(* Logix 5000 AddOnInstructionDefinition export Banner_QS18EAF_Param_v4; software revision 33.00 *)

TYPE Banner_IOL_Port_v4 :   // UDT that has all of the data items necessary to communicate with a specific Port on a IO-Link Master
STRUCT
   Port_Controlled : INT;   // Each bit represents a port on an IO-Link Master. Set to 1 to tell AOI to control that port.
   Port_Activate : INT;   // Each bit represents a port on an IO-Link Master. When ON that port will process any commands in queue.
   Port_Read : INT;   // Each bit represents a port on an IO-Link Master. Used to determine when device AOI has requested a Read command.
   Port_Write : INT;   // Each bit represents a port on an IO-Link Master. Used to determine when device AOI has requested a Write command.
   Port_RW_Complete : INT;   // Each bit represents a port on an IO-Link Master. Tells device AOI that Read or Write request has been completed.
   Port_Device_Read : INT;
   Data_Transfer : SINT[190];   // Array to transfer data from IO-Master to device AOIs.
END_STRUCT
END_TYPE

TYPE Banner_QS18EAF_RD_v4 :   // UDT that stores the Write Data for a QS18EAF.
STRUCT
   Master_Cycle_Time : INT;
   Min_Cycle_Time : INT;
   M_Sequence_Capability : INT;
   IO_Link_Version_ID : INT;
   Process_Data_Input_Length : INT;
   Process_Data_Output_Length : INT;
   Combined_Vendor_ID : DINT;   // IO-Link Vendor ID
   Vendor_ID1 : INT;
   Vendor_ID2 : INT;
   Combined_Device_ID : DINT;   // IO-Link Device ID
   Device_ID1 : INT;
   Device_ID2 : INT;
   Device_ID3 : INT;
   Serial_Number : STRING;
   Teach_State : SINT;   // 0 = Idle, 1 = SP1 Success, 4 = Wait for Command, 5 = Busy, 6 = Error.
   SP_TP1 : SINT;
   SP_TP2 : SINT;
   Current_Setpoint : DINT;   // Value in .1mm increments.
   Taught_Status : SINT;   // 0 = Not taught, 1 = Taught, 2 = Coerced to near limit, 3 = Coerced to far limit.
   All_Time_Run_Time_Counter : DINT;   // 0 to 2 Billion. 1/4 hr increments.
END_STRUCT
END_TYPE

TYPE Banner_QS18EAF_v4 :   // All of the parameters for a QS18EAF.
STRUCT
   Initial_Global_Read : BOOL;   // Determines if all of the IO-Link data has been read into the PLC yet
   Command : INT;   // Value placed in here will activate a read or write to a specifc IO-Link Index
   Read_Data : Banner_QS18EAF_RD_v4;   // Read Only Data
   Write_Data : Banner_QS18EAF_WD_v4;   // Write Data
   Archive_Data : Banner_QS18EAF_WD_v4;   // Archive Data
   Reset : BOOL;   // Resets AOI. This will force a complete parameter read of the sensor.
END_STRUCT
END_TYPE

TYPE Banner_QS18EAF_WD_v4 :   // UDT that stores the Write Data for a QS18EAF.
STRUCT
   System_Command : INT;   // See IODD file for list of commands that can be activated via the System Command interface
   Parameter_Access_Lock : SINT;   // Write access to all parameters is prohibited while value is 1. Only this parameter can be adjusted when value is 1.
   Data_Storage_Lock : SINT;   // Automatic data storage is disabled when this value is equal to 1. Read access is not affected.
   Local_Parameterization_Lock : SINT;   // Parameterization via local control elements on device is disabled.
   Local_User_Interface_Lock : SINT;   // Operation of local user interface is disabled.
   BDC1_Setpoint_SP1 : INT;   // Setpoint value in .1 mm increments.
   BDC1_Setpoint_SP2 : INT;   // Unused must be written to 0.
   BDC1_Swithpoint_Logic : INT;   // 0 = Light Operate, 1 = Dark Operate
   BDC1_BDC_Mode : INT;   // 1 = 1-Pt BGS, 128 = Object Set. Defines how the binary switching information is created depending on Setpoint parameters (SP1, SP2) and the current measurement value.
   BDC1_Hysteresis : DINT;   // Should always be 0
   BDC1_BDC_Setpoint_Selection : SINT;   // 0 = Local 1 = Remote. Controls wheater the setpoint is controlled by the POT or via the value in SP1.
   BDC1_Delay_Mode : SINT;   // 0 = Disabled, 1 = On-Off Delay, 2 = Oneshot.
   BDC1_Delay_Timer_1 : DINT;   // Range 0 to 90000. On delay or Oneshot time.
   BDC1_Delay_Timer_2 : DINT;   // Range 0 to 90000. Off delay time. If oneshot mode active this must be written as 0.
   Teach_Offset_Mode : SINT;   // 0 = Auto, 1 = User. Select between automatic tach offset and value stored in user teach offset.
   User_Teach_Offset : INT;   // User select teach offset in .1 mm increments.
   Pin_2_Configuration : SINT;   // 0 = Detection Output, 1 = Complimentary Output.
   Response_Speed : INT;   // 0 = High Speed (450 microsecond On/Off), 1 = Cross-talk (1.1 ms On/Off), 2 = Robust (1.7 ms On; 1.1 ms Off).
   Resettable_Run_Time_Counter : DINT;   // 0 to 2 Billion. 1/4 hr increments.
   All_Time_Run_Time_Event_Time : DINT;   // 0 to 2 Billion. 1/4 hr increments.
   Resettable_Run_Time_Event_Time_Counter : DINT;   // 0 to 2 Billion. 1/4 hr increments.
END_STRUCT
END_TYPE

ADD_ON_INSTRUCTION Banner_QS18EAF_Param_v4   (* revision 4.0, vendor Banner Engineering *)
// AOI to read and write parameter data to an IO-Link QS18 EAF.
VAR_IN_OUT
   QS18EAF : Banner_QS18EAF_v4; {required}
   Port_Data : Banner_IOL_Port_v4; {required}
END_VAR
VAR_INPUT
   Port : DINT; {required}
END_VAR
VAR
   Local_Control : DINT; {access None}
   Global_Read_Command_Value : INT; {access None}
   Global_Write_Command_Value : INT; {access None}
   Command_Being_Processed : BOOL; {access None}
   Update_Archive : BOOL; {access None}
   Index_Write_Inprocess : INT; {access None}
   Index_Write_Control : INT; {access None}
   Inprocess_Index : DINT; {access None}
END_VAR

ROUTINE Logic   (* ladder *)
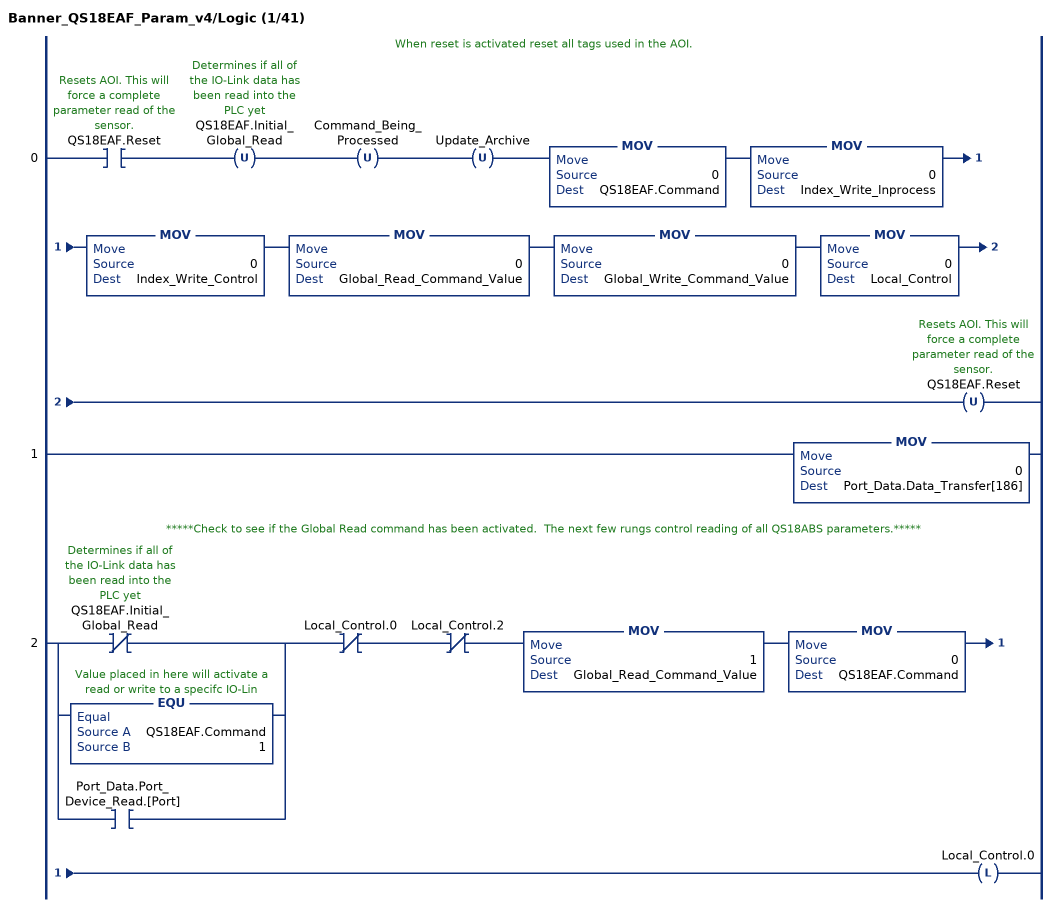
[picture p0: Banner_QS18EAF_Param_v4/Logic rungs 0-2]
   // When reset is activated reset all tags used in the AOI.
   0: XIC(QS18EAF.Reset)OTU(QS18EAF.Initial_Global_Read)OTU(Command_Being_Processed)OTU(Update_Archive)MOV(0,QS18EAF.Command)MOV(0,Index_Write_Inprocess)MOV(0,Index_Write_Control)MOV(0,Global_Read_Command_Value)MOV(0,Global_Write_Command_Value)MOV(0,Local_Control)OTU(QS18EAF.Reset);
   1: MOV(0,Port_Data.Data_Transfer[186]);
   // *****Check to see if the Global Read command has been activated.  The next few rungs control reading of all QS18ABS parameters.*****
   2: [XIO(QS18EAF.Initial_Global_Read) ,EQU(QS18EAF.Command,1) ,XIC(Port_Data.Port_Device_Read.[Port]) ]XIO(Local_Control.0)XIO(Local_Control.2)MOV(1,Global_Read_Command_Value)MOV(0,QS18EAF.Command)OTL(Local_Control.0);
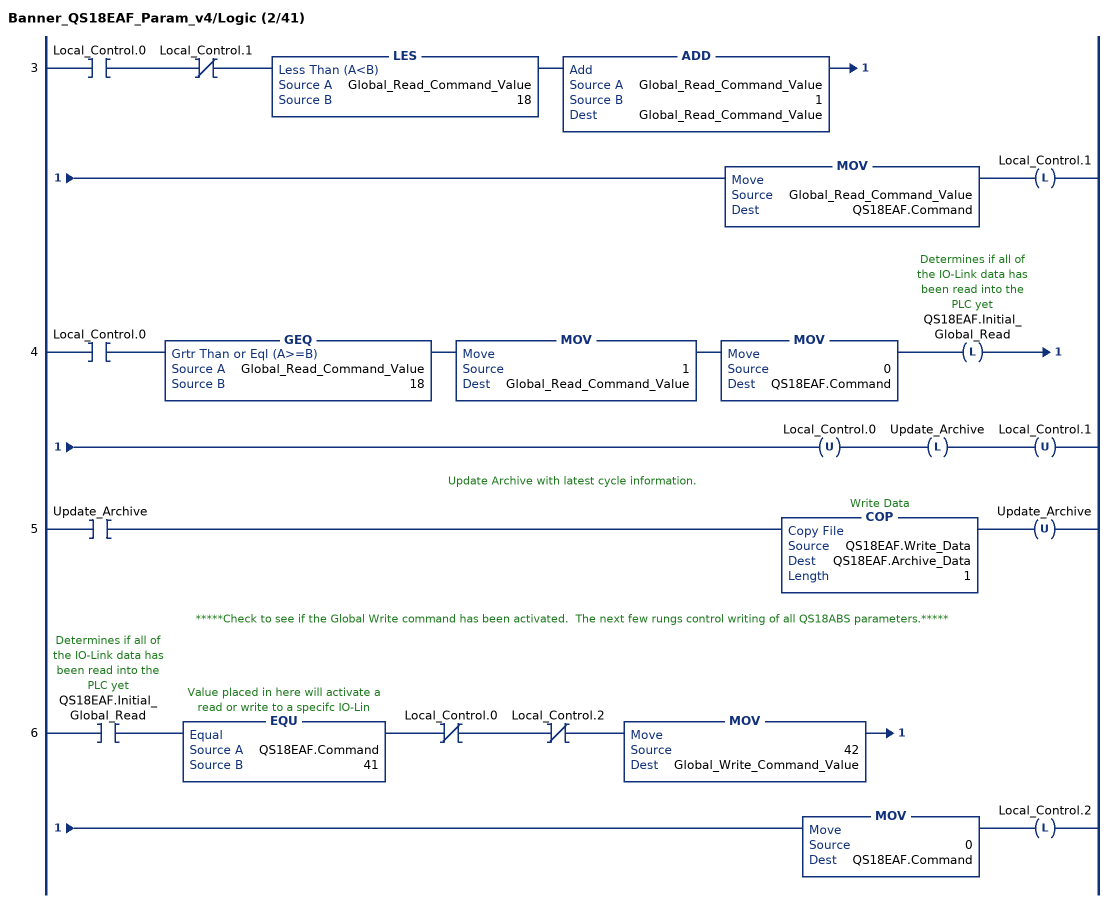
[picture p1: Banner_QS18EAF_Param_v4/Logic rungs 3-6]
   3: XIC(Local_Control.0)XIO(Local_Control.1)LES(Global_Read_Command_Value,18)ADD(Global_Read_Command_Value,1,Global_Read_Command_Value)MOV(Global_Read_Command_Value,QS18EAF.Command)OTL(Local_Control.1);
   4: XIC(Local_Control.0)GEQ(Global_Read_Command_Value,18)MOV(1,Global_Read_Command_Value)MOV(0,QS18EAF.Command)OTL(QS18EAF.Initial_Global_Read)OTU(Local_Control.0)OTL(Update_Archive)OTU(Local_Control.1);
   // Update Archive with latest cycle information.
   5: XIC(Update_Archive)COP(QS18EAF.Write_Data,QS18EAF.Archive_Data,1)OTU(Update_Archive);
   // *****Check to see if the Global Write command has been activated.  The next few rungs control writing of all QS18ABS parameters.*****
   6: XIC(QS18EAF.Initial_Global_Read)EQU(QS18EAF.Command,41)XIO(Local_Control.0)XIO(Local_Control.2)MOV(42,Global_Write_Command_Value)MOV(0,QS18EAF.Command)OTL(Local_Control.2);
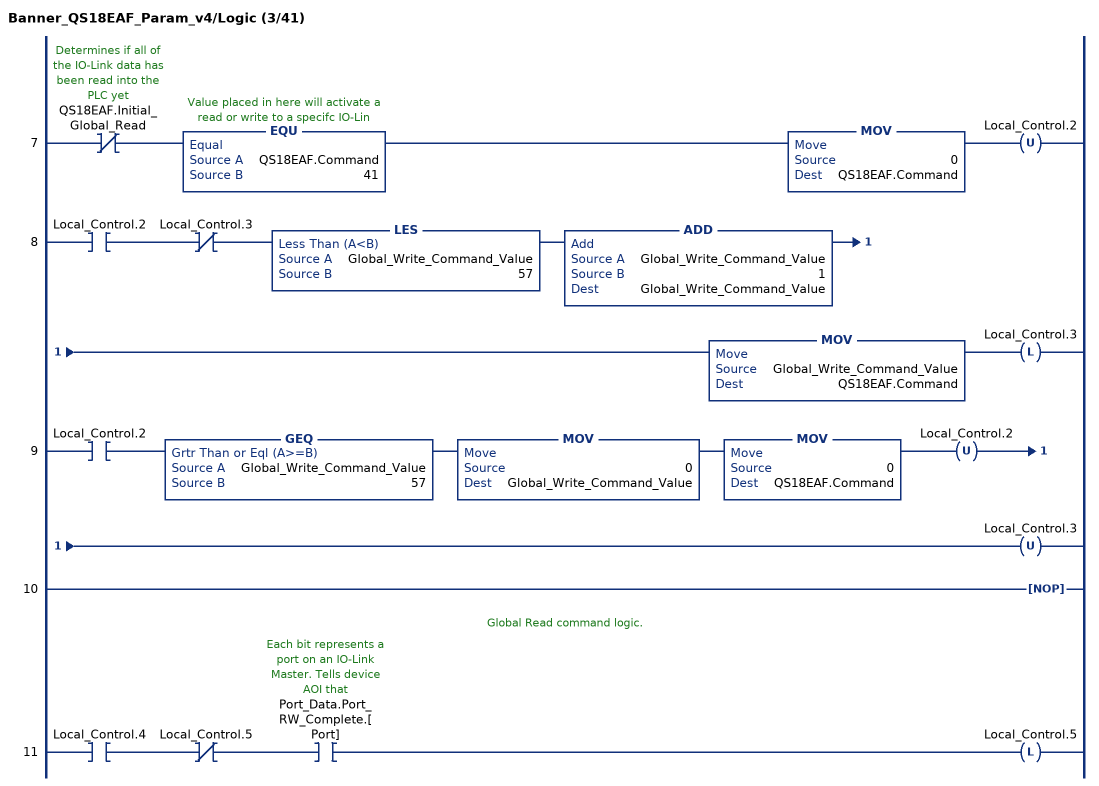
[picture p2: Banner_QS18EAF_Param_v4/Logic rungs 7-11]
   7: XIO(QS18EAF.Initial_Global_Read)EQU(QS18EAF.Command,41)MOV(0,QS18EAF.Command)OTU(Local_Control.2);
   8: XIC(Local_Control.2)XIO(Local_Control.3)LES(Global_Write_Command_Value,57)ADD(Global_Write_Command_Value,1,Global_Write_Command_Value)MOV(Global_Write_Command_Value,QS18EAF.Command)OTL(Local_Control.3);
   9: XIC(Local_Control.2)GEQ(Global_Write_Command_Value,57)MOV(0,Global_Write_Command_Value)MOV(0,QS18EAF.Command)OTU(Local_Control.2)OTU(Local_Control.3);
   10: NOP();
   // Global Read command logic.
   11: XIC(Local_Control.4)XIO(Local_Control.5)XIC(Port_Data.Port_RW_Complete.[Port])OTL(Local_Control.5);
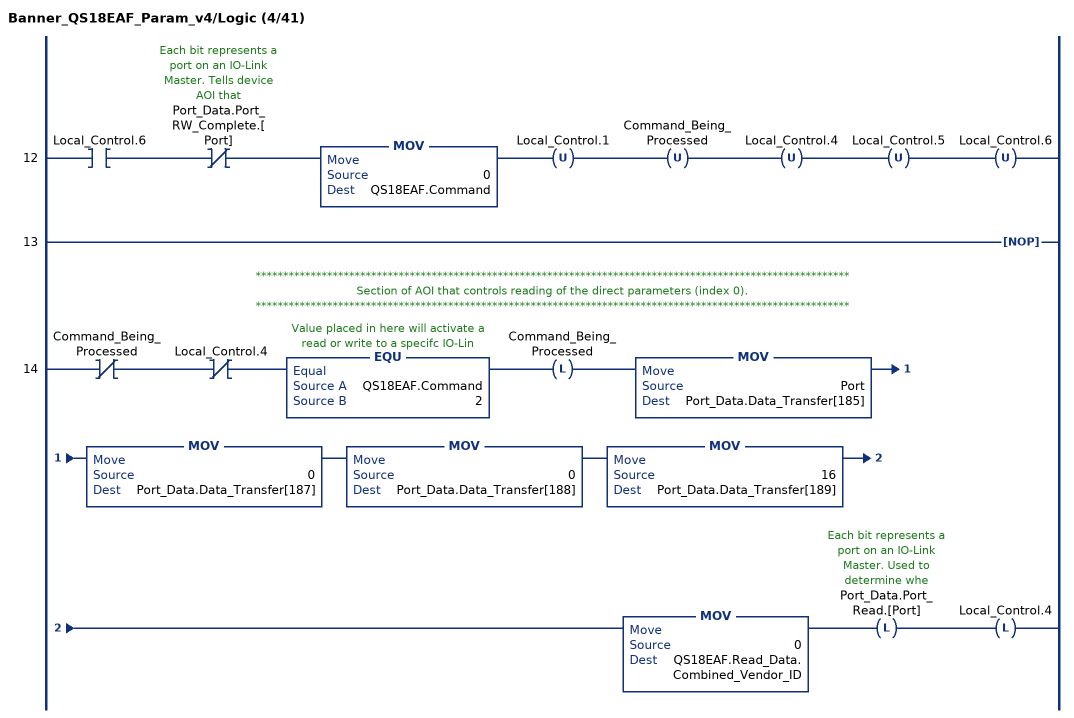
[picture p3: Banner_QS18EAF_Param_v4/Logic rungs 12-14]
   12: XIC(Local_Control.6)XIO(Port_Data.Port_RW_Complete.[Port])MOV(0,QS18EAF.Command)OTU(Local_Control.1)OTU(Command_Being_Processed)OTU(Local_Control.4)OTU(Local_Control.5)OTU(Local_Control.6);
   13: NOP();
   // ************************************************************************************************************
   // Section of AOI that controls reading of the direct parameters (index 0).
   // ************************************************************************************************************
   14: XIO(Command_Being_Processed)XIO(Local_Control.4)EQU(QS18EAF.Command,2)OTL(Command_Being_Processed)MOV(Port,Port_Data.Data_Transfer[185])MOV(0,Port_Data.Data_Transfer[187])MOV(0,Port_Data.Data_Transfer[188])MOV(16,Port_Data.Data_Transfer[189])MOV(0,QS18EAF.Read_Data.Combined_Vendor_ID)OTL(Port_Data.Port_Read.[Port])OTL(Local_Control.4);
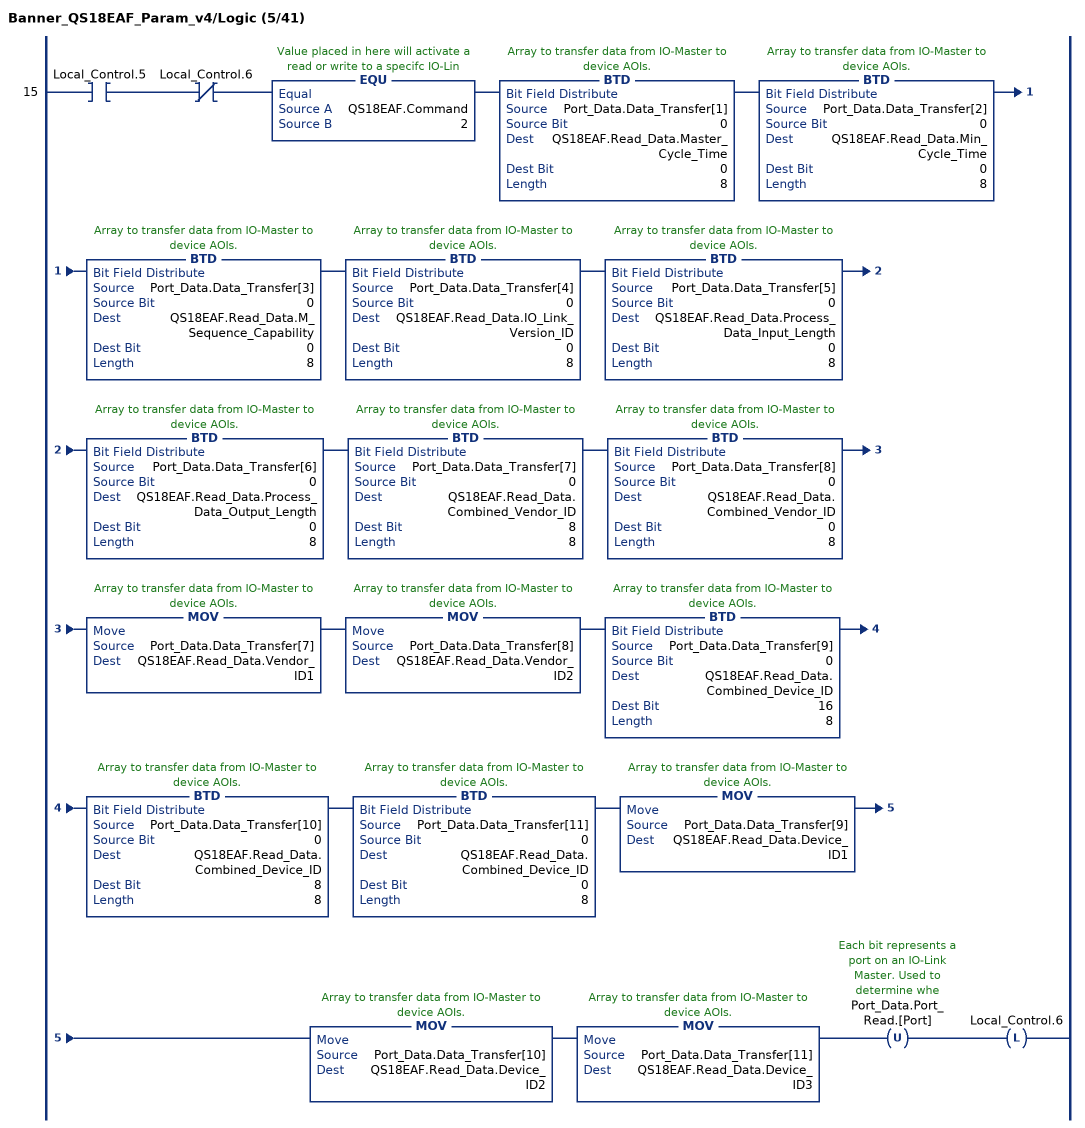
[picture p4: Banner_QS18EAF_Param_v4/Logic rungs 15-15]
   15: XIC(Local_Control.5)XIO(Local_Control.6)EQU(QS18EAF.Command,2)BTD(Port_Data.Data_Transfer[1],0,QS18EAF.Read_Data.Master_Cycle_Time,0,8)BTD(Port_Data.Data_Transfer[2],0,QS18EAF.Read_Data.Min_Cycle_Time,0,8)BTD(Port_Data.Data_Transfer[3],0,QS18EAF.Read_Data.M_Sequence_Capability,0,8)BTD(Port_Data.Data_Transfer[4],0,QS18EAF.Read_Data.IO_Link_Version_ID,0,8)BTD(Port_Data.Data_Transfer[5],0,QS18EAF.Read_Data.Process_Data_Input_Length,0,8)BTD(Port_Data.Data_Transfer[6],0,QS18EAF.Read_Data.Process_Data_Output_Length,0,8)BTD(Port_Data.Data_Transfer[7],0,QS18EAF.Read_Data.Combined_Vendor_ID,8,8)BTD(Port_Data.Data_Transfer[8],0,QS18EAF.Read_Data.Combined_Vendor_ID,0,8)MOV(Port_Data.Data_Transfer[7],QS18EAF.Read_Data.Vendor_ID1)MOV(Port_Data.Data_Transfer[8],QS18EAF.Read_Data.Vendor_ID2)BTD(Port_Data.Data_Transfer[9],0,QS18EAF.Read_Data.Combined_Device_ID,16,8)BTD(Port_Data.Data_Transfer[10],0,QS18EAF.Read_Data.Combined_Device_ID,8,8)BTD(Port_Data.Data_Transfer[11],0,QS18EAF.Read_Data.Combined_Device_ID,0,8)MOV(Port_Data.Data_Transfer[9],QS18EAF.Read_Data.Device_ID1)MOV(Port_Data.Data_Transfer[10],QS18EAF.Read_Data.Device_ID2)MOV(Port_Data.Data_Transfer[11],QS18EAF.Read_Data.Device_ID3)OTU(Port_Data.Port_Read.[Port])OTL(Local_Control.6);
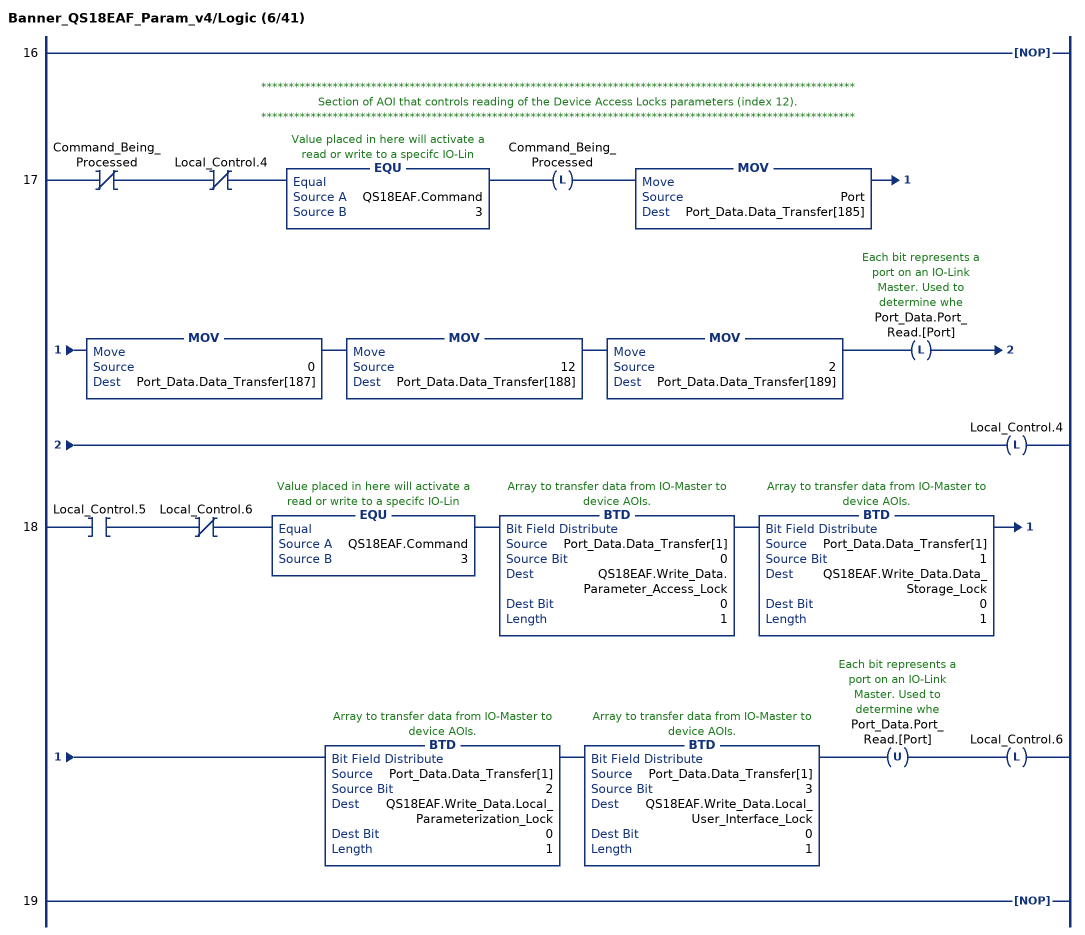
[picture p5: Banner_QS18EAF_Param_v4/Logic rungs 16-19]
   16: NOP();
   // ************************************************************************************************************
   // Section of AOI that controls reading of the Device Access Locks parameters (index 12).
   // ************************************************************************************************************
   17: XIO(Command_Being_Processed)XIO(Local_Control.4)EQU(QS18EAF.Command,3)OTL(Command_Being_Processed)MOV(Port,Port_Data.Data_Transfer[185])MOV(0,Port_Data.Data_Transfer[187])MOV(12,Port_Data.Data_Transfer[188])MOV(2,Port_Data.Data_Transfer[189])OTL(Port_Data.Port_Read.[Port])OTL(Local_Control.4);
   18: XIC(Local_Control.5)XIO(Local_Control.6)EQU(QS18EAF.Command,3)BTD(Port_Data.Data_Transfer[1],0,QS18EAF.Write_Data.Parameter_Access_Lock,0,1)BTD(Port_Data.Data_Transfer[1],1,QS18EAF.Write_Data.Data_Storage_Lock,0,1)BTD(Port_Data.Data_Transfer[1],2,QS18EAF.Write_Data.Local_Parameterization_Lock,0,1)BTD(Port_Data.Data_Transfer[1],3,QS18EAF.Write_Data.Local_User_Interface_Lock,0,1)OTU(Port_Data.Port_Read.[Port])OTL(Local_Control.6);
   19: NOP();
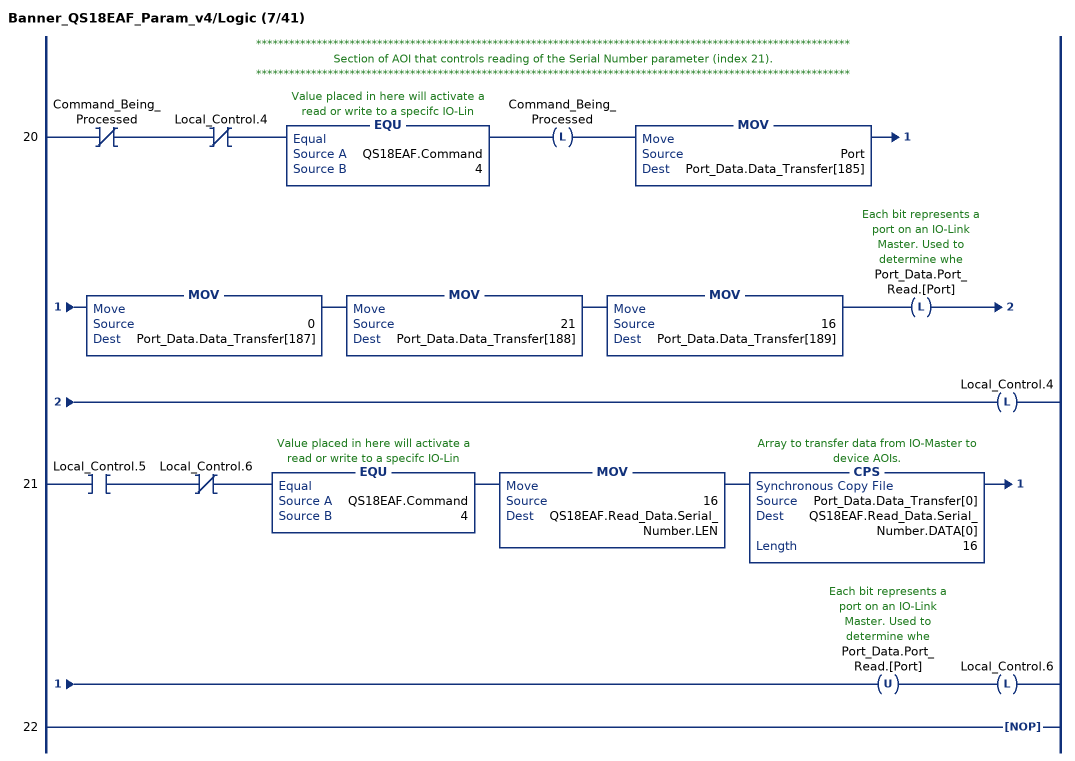
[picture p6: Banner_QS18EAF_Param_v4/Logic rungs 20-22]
   // ************************************************************************************************************
   // Section of AOI that controls reading of the Serial Number parameter (index 21).
   // ************************************************************************************************************
   20: XIO(Command_Being_Processed)XIO(Local_Control.4)EQU(QS18EAF.Command,4)OTL(Command_Being_Processed)MOV(Port,Port_Data.Data_Transfer[185])MOV(0,Port_Data.Data_Transfer[187])MOV(21,Port_Data.Data_Transfer[188])MOV(16,Port_Data.Data_Transfer[189])OTL(Port_Data.Port_Read.[Port])OTL(Local_Control.4);
   21: XIC(Local_Control.5)XIO(Local_Control.6)EQU(QS18EAF.Command,4)MOV(16,QS18EAF.Read_Data.Serial_Number.LEN)CPS(Port_Data.Data_Transfer[0],QS18EAF.Read_Data.Serial_Number.DATA[0],16)OTU(Port_Data.Port_Read.[Port])OTL(Local_Control.6);
   22: NOP();
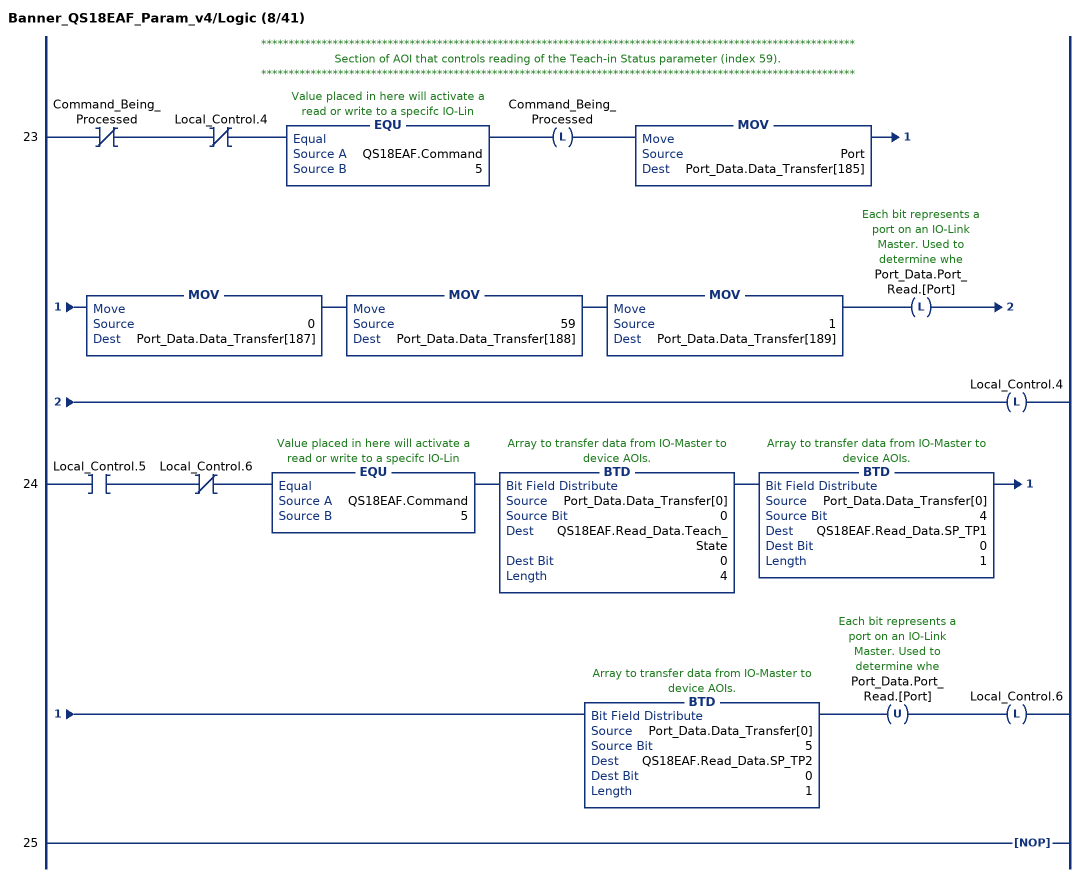
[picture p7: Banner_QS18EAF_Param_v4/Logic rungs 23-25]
   // ************************************************************************************************************
   // Section of AOI that controls reading of the Teach-in Status parameter (index 59).
   // ************************************************************************************************************
   23: XIO(Command_Being_Processed)XIO(Local_Control.4)EQU(QS18EAF.Command,5)OTL(Command_Being_Processed)MOV(Port,Port_Data.Data_Transfer[185])MOV(0,Port_Data.Data_Transfer[187])MOV(59,Port_Data.Data_Transfer[188])MOV(1,Port_Data.Data_Transfer[189])OTL(Port_Data.Port_Read.[Port])OTL(Local_Control.4);
   24: XIC(Local_Control.5)XIO(Local_Control.6)EQU(QS18EAF.Command,5)BTD(Port_Data.Data_Transfer[0],0,QS18EAF.Read_Data.Teach_State,0,4)BTD(Port_Data.Data_Transfer[0],4,QS18EAF.Read_Data.SP_TP1,0,1)BTD(Port_Data.Data_Transfer[0],5,QS18EAF.Read_Data.SP_TP2,0,1)OTU(Port_Data.Port_Read.[Port])OTL(Local_Control.6);
   25: NOP();
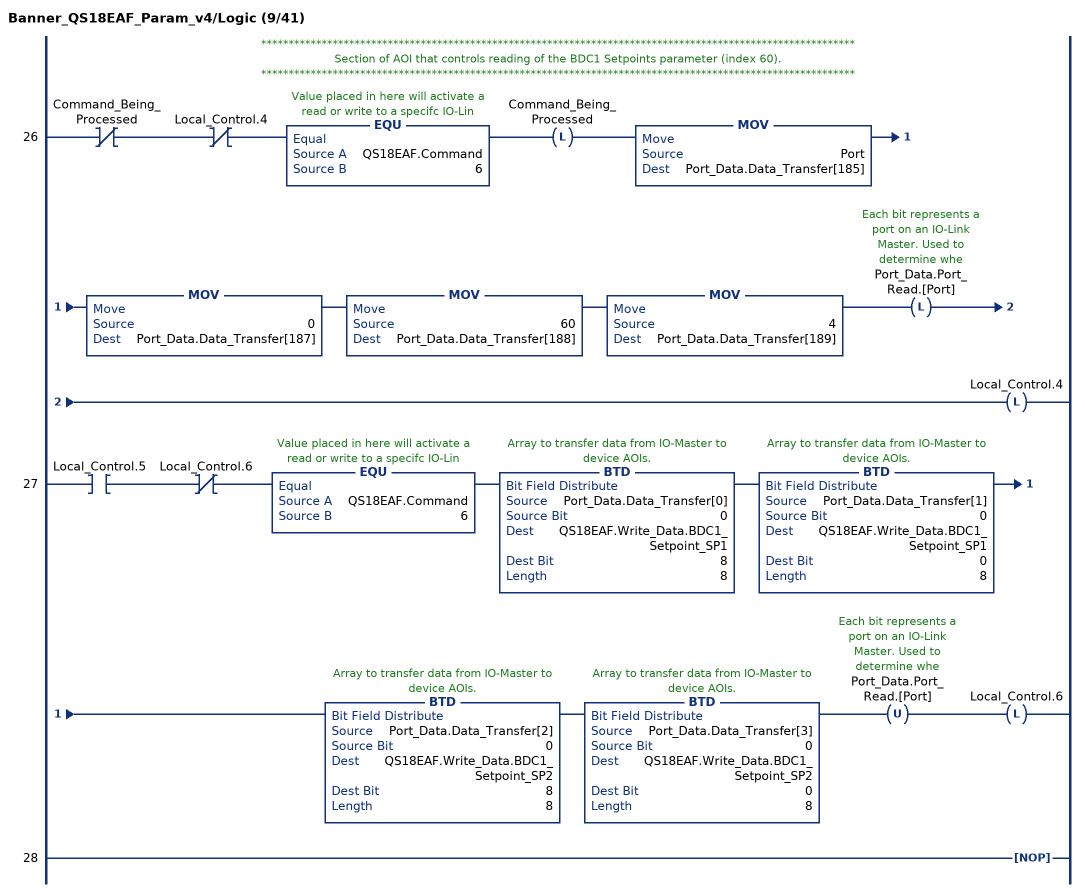
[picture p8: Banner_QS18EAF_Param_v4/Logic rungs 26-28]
   // ************************************************************************************************************
   // Section of AOI that controls reading of the BDC1 Setpoints parameter (index 60).
   // ************************************************************************************************************
   26: XIO(Command_Being_Processed)XIO(Local_Control.4)EQU(QS18EAF.Command,6)OTL(Command_Being_Processed)MOV(Port,Port_Data.Data_Transfer[185])MOV(0,Port_Data.Data_Transfer[187])MOV(60,Port_Data.Data_Transfer[188])MOV(4,Port_Data.Data_Transfer[189])OTL(Port_Data.Port_Read.[Port])OTL(Local_Control.4);
   27: XIC(Local_Control.5)XIO(Local_Control.6)EQU(QS18EAF.Command,6)BTD(Port_Data.Data_Transfer[0],0,QS18EAF.Write_Data.BDC1_Setpoint_SP1,8,8)BTD(Port_Data.Data_Transfer[1],0,QS18EAF.Write_Data.BDC1_Setpoint_SP1,0,8)BTD(Port_Data.Data_Transfer[2],0,QS18EAF.Write_Data.BDC1_Setpoint_SP2,8,8)BTD(Port_Data.Data_Transfer[3],0,QS18EAF.Write_Data.BDC1_Setpoint_SP2,0,8)OTU(Port_Data.Port_Read.[Port])OTL(Local_Control.6);
   28: NOP();
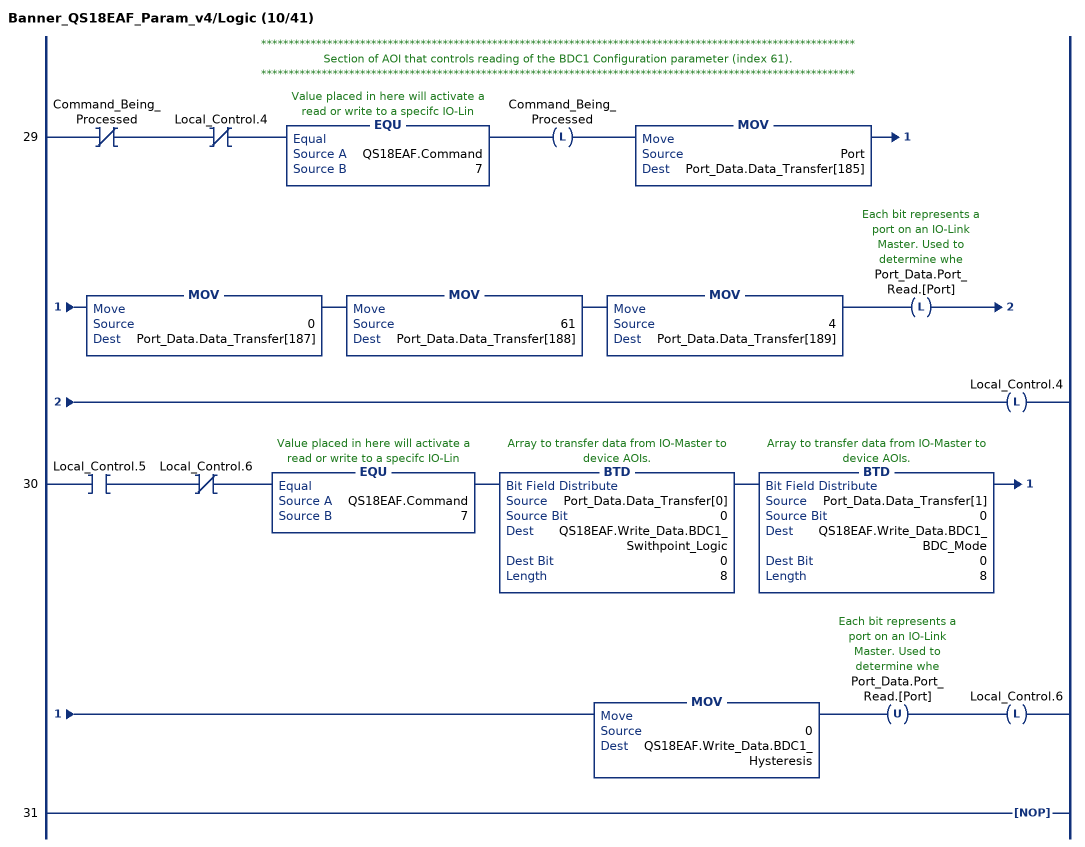
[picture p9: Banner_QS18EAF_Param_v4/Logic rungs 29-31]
   // ************************************************************************************************************
   // Section of AOI that controls reading of the BDC1 Configuration parameter (index 61).
   // ************************************************************************************************************
   29: XIO(Command_Being_Processed)XIO(Local_Control.4)EQU(QS18EAF.Command,7)OTL(Command_Being_Processed)MOV(Port,Port_Data.Data_Transfer[185])MOV(0,Port_Data.Data_Transfer[187])MOV(61,Port_Data.Data_Transfer[188])MOV(4,Port_Data.Data_Transfer[189])OTL(Port_Data.Port_Read.[Port])OTL(Local_Control.4);
   30: XIC(Local_Control.5)XIO(Local_Control.6)EQU(QS18EAF.Command,7)BTD(Port_Data.Data_Transfer[0],0,QS18EAF.Write_Data.BDC1_Swithpoint_Logic,0,8)BTD(Port_Data.Data_Transfer[1],0,QS18EAF.Write_Data.BDC1_BDC_Mode,0,8)MOV(0,QS18EAF.Write_Data.BDC1_Hysteresis)OTU(Port_Data.Port_Read.[Port])OTL(Local_Control.6);
   31: NOP();
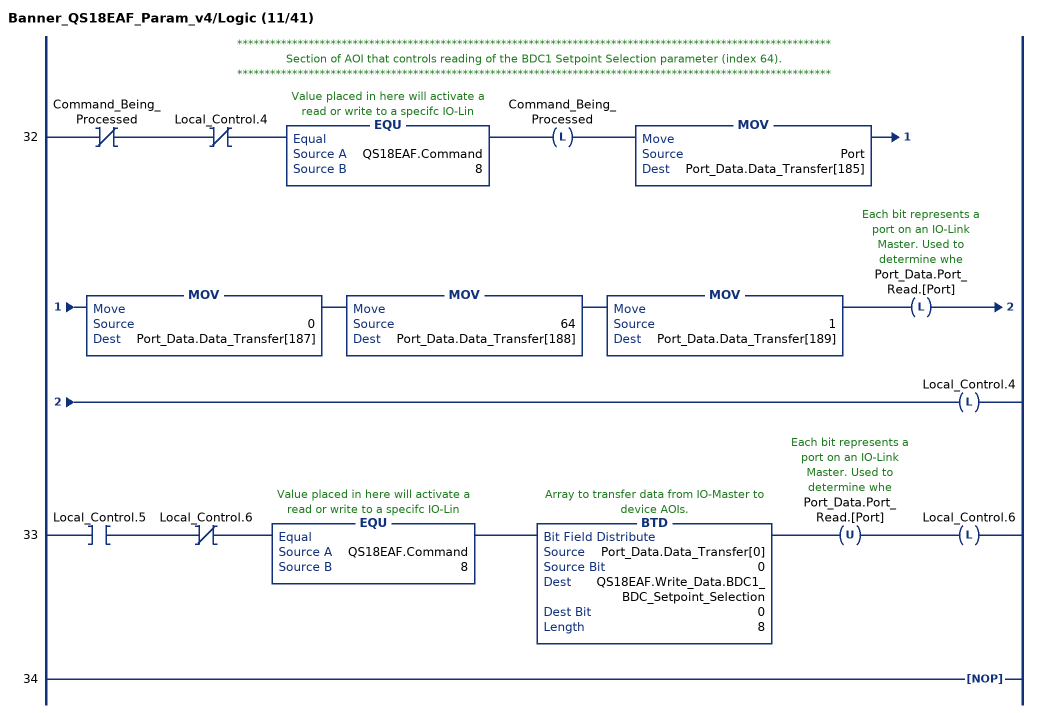
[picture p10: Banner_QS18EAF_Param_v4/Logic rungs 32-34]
   // ************************************************************************************************************
   // Section of AOI that controls reading of the BDC1 Setpoint Selection parameter (index 64).
   // ************************************************************************************************************
   32: XIO(Command_Being_Processed)XIO(Local_Control.4)EQU(QS18EAF.Command,8)OTL(Command_Being_Processed)MOV(Port,Port_Data.Data_Transfer[185])MOV(0,Port_Data.Data_Transfer[187])MOV(64,Port_Data.Data_Transfer[188])MOV(1,Port_Data.Data_Transfer[189])OTL(Port_Data.Port_Read.[Port])OTL(Local_Control.4);
   33: XIC(Local_Control.5)XIO(Local_Control.6)EQU(QS18EAF.Command,8)BTD(Port_Data.Data_Transfer[0],0,QS18EAF.Write_Data.BDC1_BDC_Setpoint_Selection,0,8)OTU(Port_Data.Port_Read.[Port])OTL(Local_Control.6);
   34: NOP();
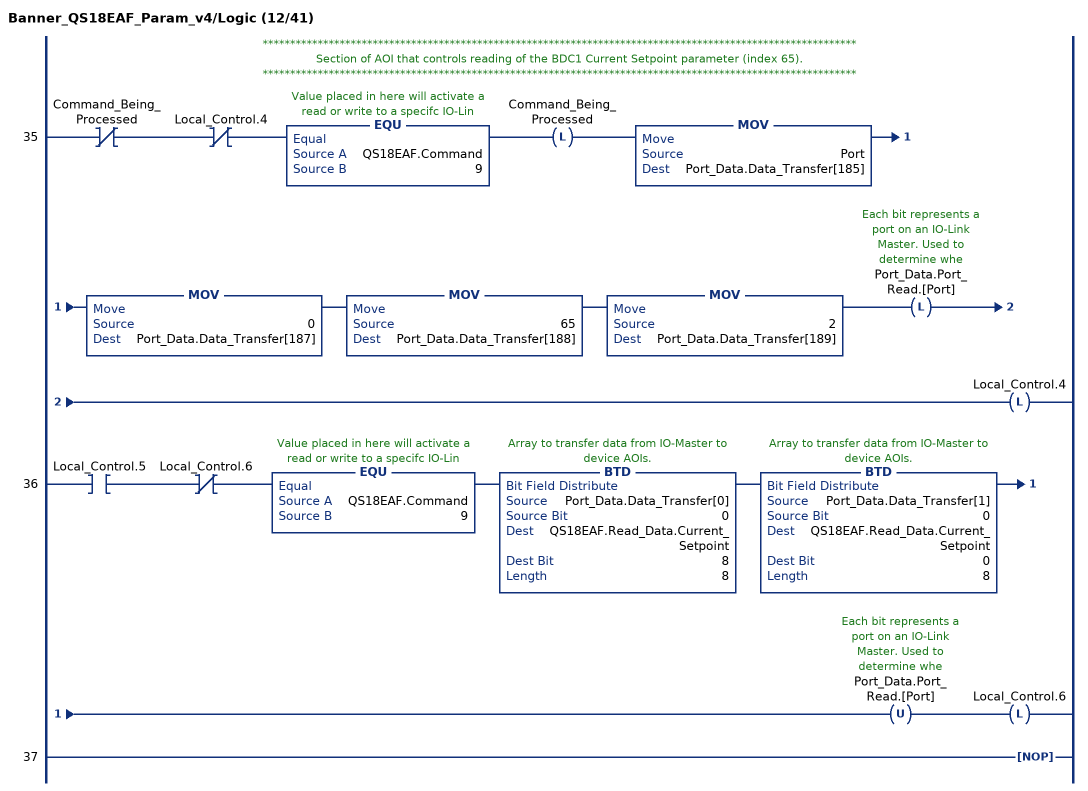
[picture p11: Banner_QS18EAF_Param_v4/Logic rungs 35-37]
   // ************************************************************************************************************
   // Section of AOI that controls reading of the BDC1 Current Setpoint parameter (index 65).
   // ************************************************************************************************************
   35: XIO(Command_Being_Processed)XIO(Local_Control.4)EQU(QS18EAF.Command,9)OTL(Command_Being_Processed)MOV(Port,Port_Data.Data_Transfer[185])MOV(0,Port_Data.Data_Transfer[187])MOV(65,Port_Data.Data_Transfer[188])MOV(2,Port_Data.Data_Transfer[189])OTL(Port_Data.Port_Read.[Port])OTL(Local_Control.4);
   36: XIC(Local_Control.5)XIO(Local_Control.6)EQU(QS18EAF.Command,9)BTD(Port_Data.Data_Transfer[0],0,QS18EAF.Read_Data.Current_Setpoint,8,8)BTD(Port_Data.Data_Transfer[1],0,QS18EAF.Read_Data.Current_Setpoint,0,8)OTU(Port_Data.Port_Read.[Port])OTL(Local_Control.6);
   37: NOP();
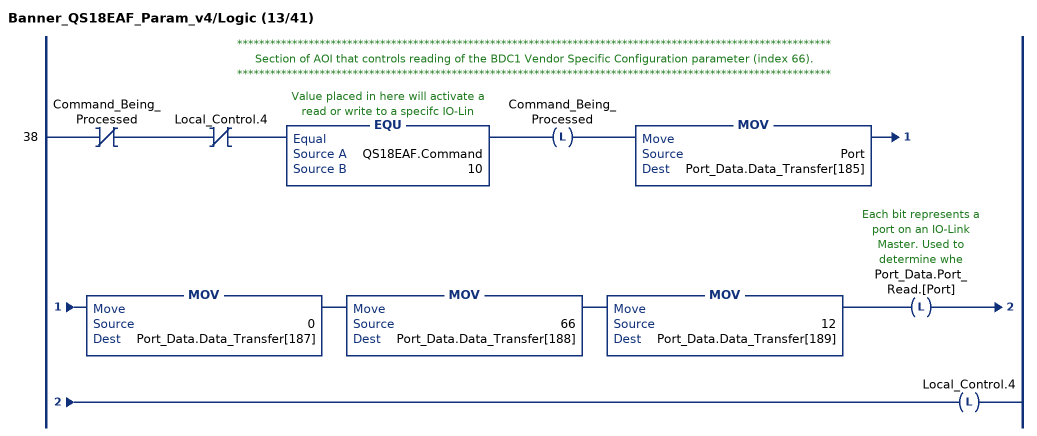
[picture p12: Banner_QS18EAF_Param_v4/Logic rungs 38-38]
   // ************************************************************************************************************
   // Section of AOI that controls reading of the BDC1 Vendor Specific Configuration parameter (index 66).
   // ************************************************************************************************************
   38: XIO(Command_Being_Processed)XIO(Local_Control.4)EQU(QS18EAF.Command,10)OTL(Command_Being_Processed)MOV(Port,Port_Data.Data_Transfer[185])MOV(0,Port_Data.Data_Transfer[187])MOV(66,Port_Data.Data_Transfer[188])MOV(12,Port_Data.Data_Transfer[189])OTL(Port_Data.Port_Read.[Port])OTL(Local_Control.4);
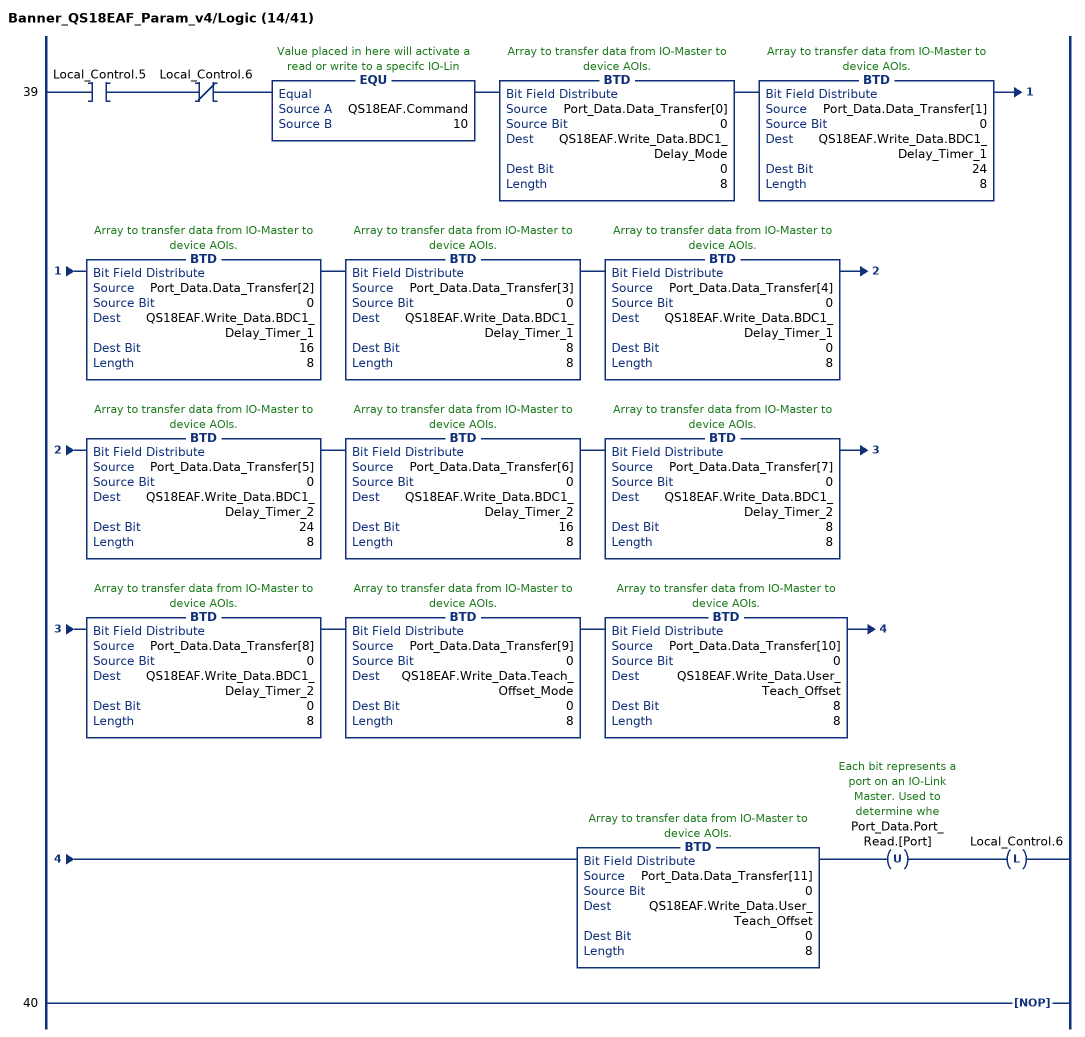
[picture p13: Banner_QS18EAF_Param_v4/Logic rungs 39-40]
   39: XIC(Local_Control.5)XIO(Local_Control.6)EQU(QS18EAF.Command,10)BTD(Port_Data.Data_Transfer[0],0,QS18EAF.Write_Data.BDC1_Delay_Mode,0,8)BTD(Port_Data.Data_Transfer[1],0,QS18EAF.Write_Data.BDC1_Delay_Timer_1,24,8)BTD(Port_Data.Data_Transfer[2],0,QS18EAF.Write_Data.BDC1_Delay_Timer_1,16,8)BTD(Port_Data.Data_Transfer[3],0,QS18EAF.Write_Data.BDC1_Delay_Timer_1,8,8)BTD(Port_Data.Data_Transfer[4],0,QS18EAF.Write_Data.BDC1_Delay_Timer_1,0,8)BTD(Port_Data.Data_Transfer[5],0,QS18EAF.Write_Data.BDC1_Delay_Timer_2,24,8)BTD(Port_Data.Data_Transfer[6],0,QS18EAF.Write_Data.BDC1_Delay_Timer_2,16,8)BTD(Port_Data.Data_Transfer[7],0,QS18EAF.Write_Data.BDC1_Delay_Timer_2,8,8)BTD(Port_Data.Data_Transfer[8],0,QS18EAF.Write_Data.BDC1_Delay_Timer_2,0,8)BTD(Port_Data.Data_Transfer[9],0,QS18EAF.Write_Data.Teach_Offset_Mode,0,8)BTD(Port_Data.Data_Transfer[10],0,QS18EAF.Write_Data.User_Teach_Offset,8,8)BTD(Port_Data.Data_Transfer[11],0,QS18EAF.Write_Data.User_Teach_Offset,0,8)OTU(Port_Data.Port_Read.[Port])OTL(Local_Control.6);
   40: NOP();
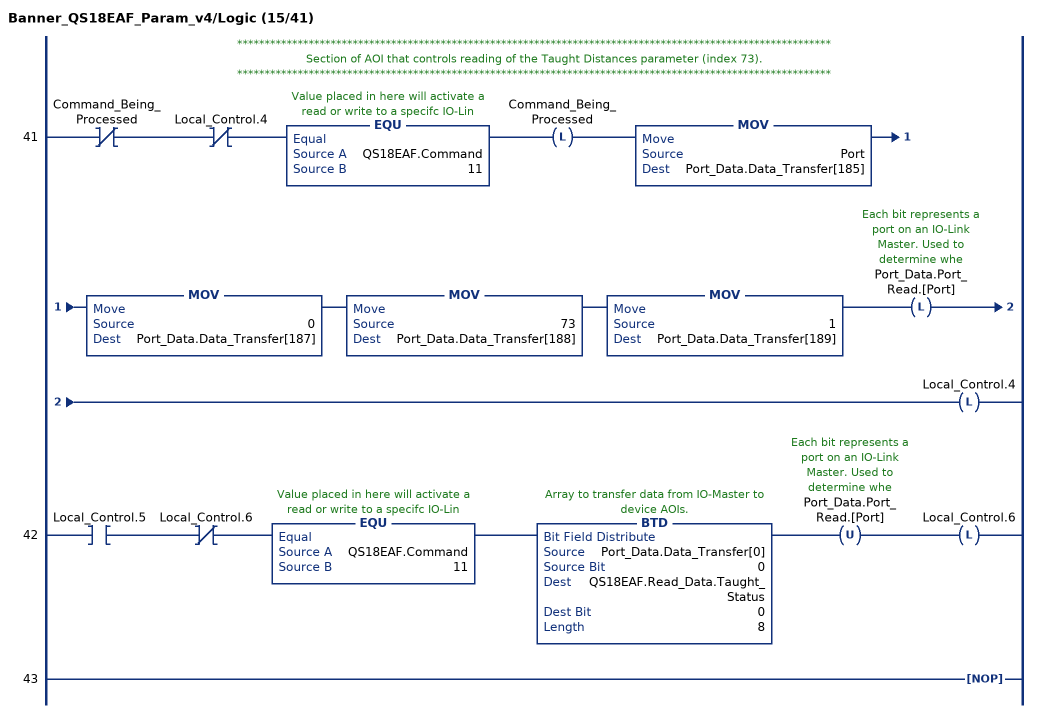
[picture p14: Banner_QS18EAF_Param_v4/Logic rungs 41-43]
   // ************************************************************************************************************
   // Section of AOI that controls reading of the Taught Distances parameter (index 73).
   // ************************************************************************************************************
   41: XIO(Command_Being_Processed)XIO(Local_Control.4)EQU(QS18EAF.Command,11)OTL(Command_Being_Processed)MOV(Port,Port_Data.Data_Transfer[185])MOV(0,Port_Data.Data_Transfer[187])MOV(73,Port_Data.Data_Transfer[188])MOV(1,Port_Data.Data_Transfer[189])OTL(Port_Data.Port_Read.[Port])OTL(Local_Control.4);
   42: XIC(Local_Control.5)XIO(Local_Control.6)EQU(QS18EAF.Command,11)BTD(Port_Data.Data_Transfer[0],0,QS18EAF.Read_Data.Taught_Status,0,8)OTU(Port_Data.Port_Read.[Port])OTL(Local_Control.6);
   43: NOP();
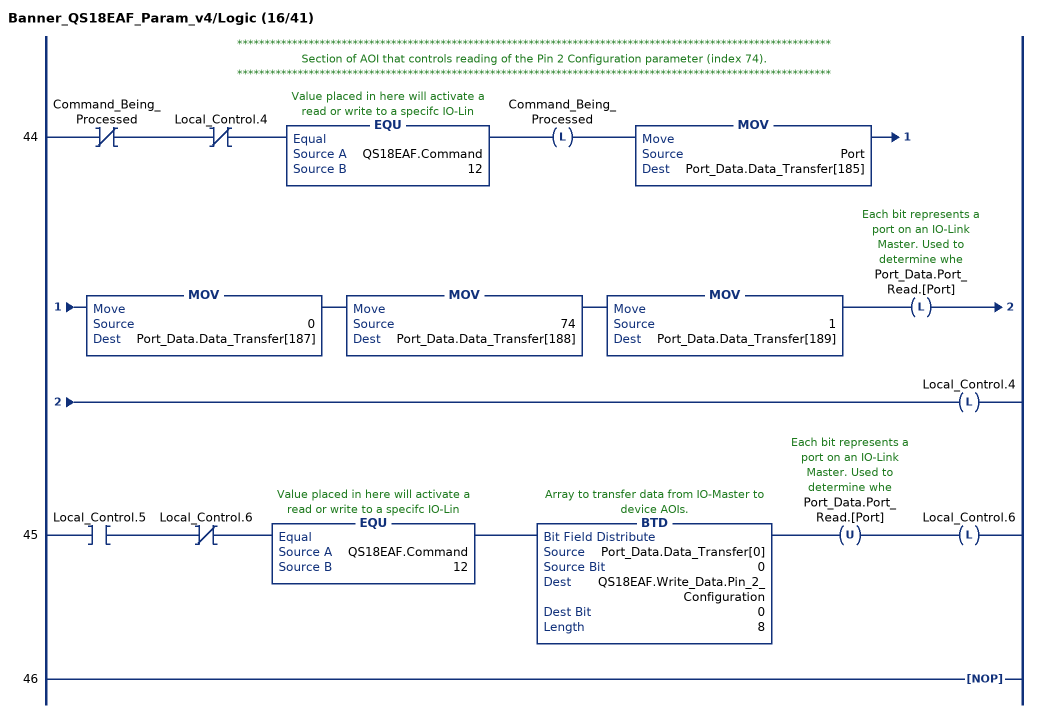
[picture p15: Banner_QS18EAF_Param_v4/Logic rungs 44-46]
   // ************************************************************************************************************
   // Section of AOI that controls reading of the Pin 2 Configuration parameter (index 74).
   // ************************************************************************************************************
   44: XIO(Command_Being_Processed)XIO(Local_Control.4)EQU(QS18EAF.Command,12)OTL(Command_Being_Processed)MOV(Port,Port_Data.Data_Transfer[185])MOV(0,Port_Data.Data_Transfer[187])MOV(74,Port_Data.Data_Transfer[188])MOV(1,Port_Data.Data_Transfer[189])OTL(Port_Data.Port_Read.[Port])OTL(Local_Control.4);
   45: XIC(Local_Control.5)XIO(Local_Control.6)EQU(QS18EAF.Command,12)BTD(Port_Data.Data_Transfer[0],0,QS18EAF.Write_Data.Pin_2_Configuration,0,8)OTU(Port_Data.Port_Read.[Port])OTL(Local_Control.6);
   46: NOP();
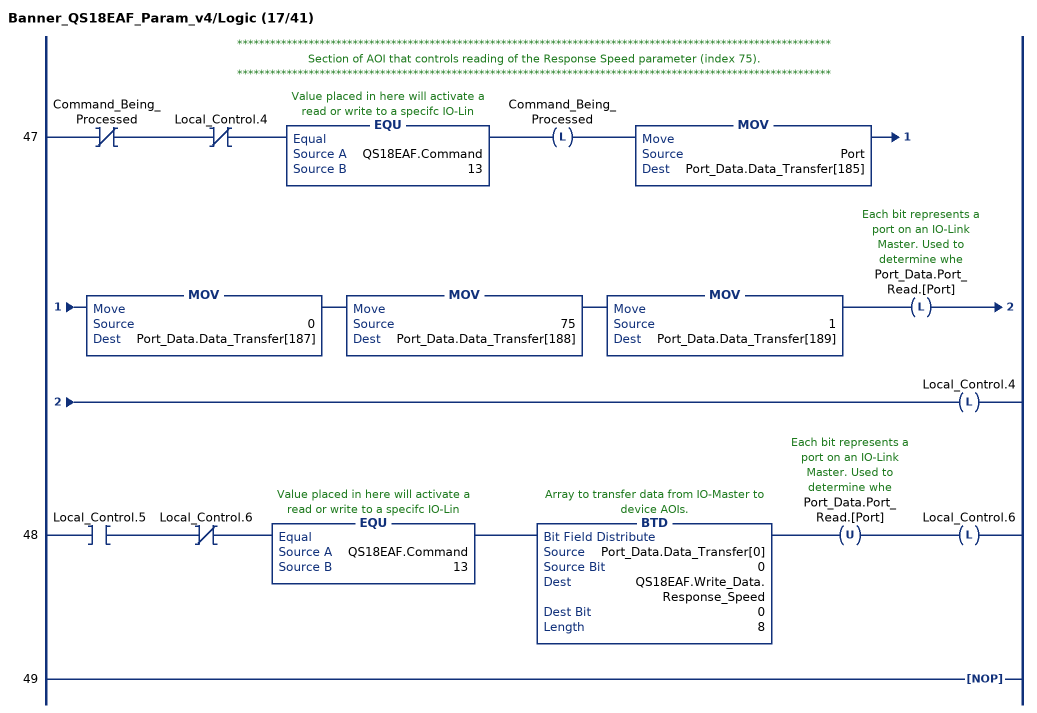
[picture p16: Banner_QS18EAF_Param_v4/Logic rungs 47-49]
   // ************************************************************************************************************
   // Section of AOI that controls reading of the Response Speed parameter (index 75).
   // ************************************************************************************************************
   47: XIO(Command_Being_Processed)XIO(Local_Control.4)EQU(QS18EAF.Command,13)OTL(Command_Being_Processed)MOV(Port,Port_Data.Data_Transfer[185])MOV(0,Port_Data.Data_Transfer[187])MOV(75,Port_Data.Data_Transfer[188])MOV(1,Port_Data.Data_Transfer[189])OTL(Port_Data.Port_Read.[Port])OTL(Local_Control.4);
   48: XIC(Local_Control.5)XIO(Local_Control.6)EQU(QS18EAF.Command,13)BTD(Port_Data.Data_Transfer[0],0,QS18EAF.Write_Data.Response_Speed,0,8)OTU(Port_Data.Port_Read.[Port])OTL(Local_Control.6);
   49: NOP();
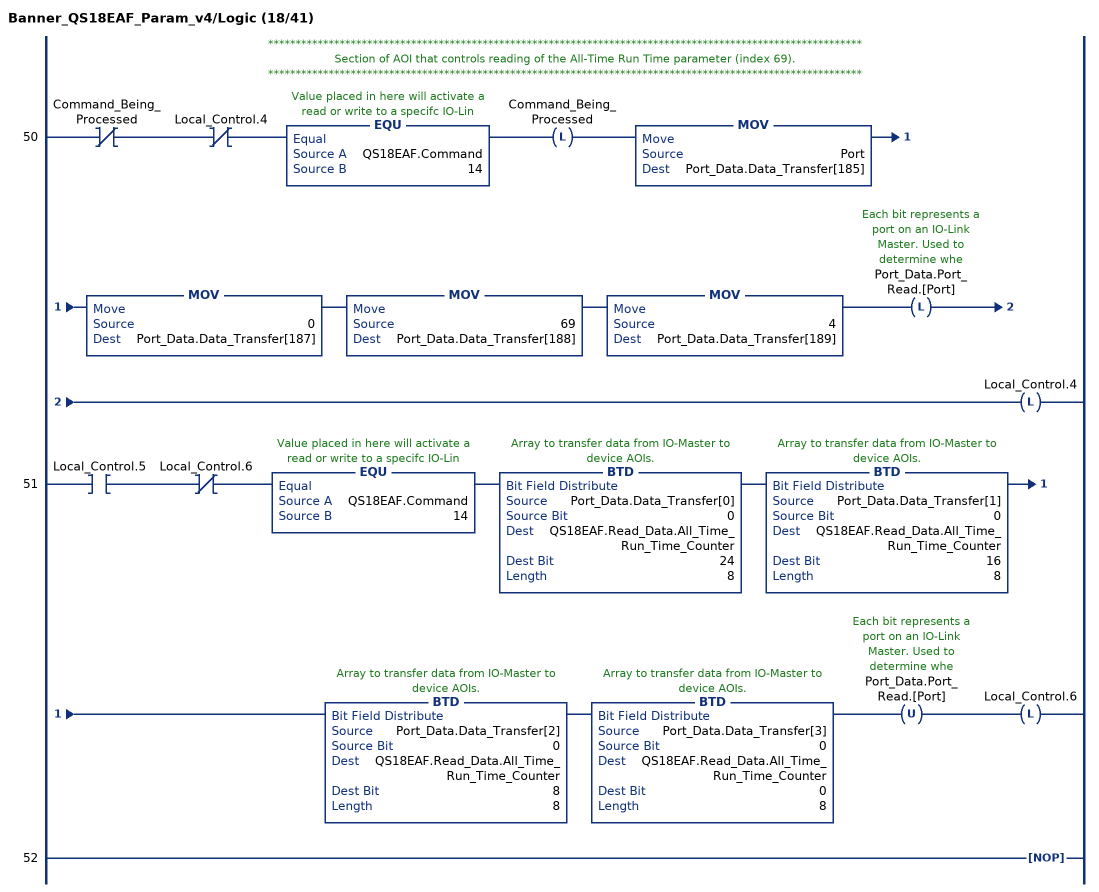
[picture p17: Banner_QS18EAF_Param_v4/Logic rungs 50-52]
   // ************************************************************************************************************
   // Section of AOI that controls reading of the All-Time Run Time parameter (index 69).
   // ************************************************************************************************************
   50: XIO(Command_Being_Processed)XIO(Local_Control.4)EQU(QS18EAF.Command,14)OTL(Command_Being_Processed)MOV(Port,Port_Data.Data_Transfer[185])MOV(0,Port_Data.Data_Transfer[187])MOV(69,Port_Data.Data_Transfer[188])MOV(4,Port_Data.Data_Transfer[189])OTL(Port_Data.Port_Read.[Port])OTL(Local_Control.4);
   51: XIC(Local_Control.5)XIO(Local_Control.6)EQU(QS18EAF.Command,14)BTD(Port_Data.Data_Transfer[0],0,QS18EAF.Read_Data.All_Time_Run_Time_Counter,24,8)BTD(Port_Data.Data_Transfer[1],0,QS18EAF.Read_Data.All_Time_Run_Time_Counter,16,8)BTD(Port_Data.Data_Transfer[2],0,QS18EAF.Read_Data.All_Time_Run_Time_Counter,8,8)BTD(Port_Data.Data_Transfer[3],0,QS18EAF.Read_Data.All_Time_Run_Time_Counter,0,8)OTU(Port_Data.Port_Read.[Port])OTL(Local_Control.6);
   52: NOP();
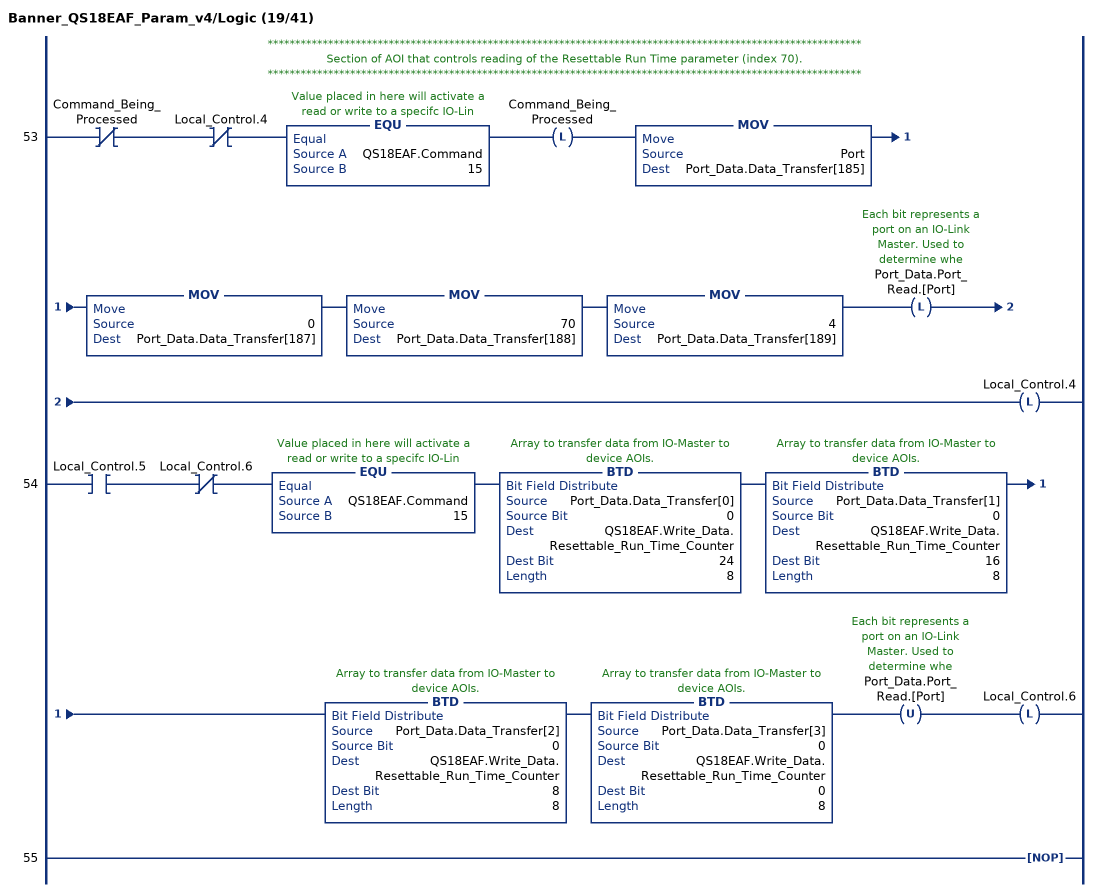
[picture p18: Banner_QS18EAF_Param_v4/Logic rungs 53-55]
   // ************************************************************************************************************
   // Section of AOI that controls reading of the Resettable Run Time parameter (index 70).
   // ************************************************************************************************************
   53: XIO(Command_Being_Processed)XIO(Local_Control.4)EQU(QS18EAF.Command,15)OTL(Command_Being_Processed)MOV(Port,Port_Data.Data_Transfer[185])MOV(0,Port_Data.Data_Transfer[187])MOV(70,Port_Data.Data_Transfer[188])MOV(4,Port_Data.Data_Transfer[189])OTL(Port_Data.Port_Read.[Port])OTL(Local_Control.4);
   54: XIC(Local_Control.5)XIO(Local_Control.6)EQU(QS18EAF.Command,15)BTD(Port_Data.Data_Transfer[0],0,QS18EAF.Write_Data.Resettable_Run_Time_Counter,24,8)BTD(Port_Data.Data_Transfer[1],0,QS18EAF.Write_Data.Resettable_Run_Time_Counter,16,8)BTD(Port_Data.Data_Transfer[2],0,QS18EAF.Write_Data.Resettable_Run_Time_Counter,8,8)BTD(Port_Data.Data_Transfer[3],0,QS18EAF.Write_Data.Resettable_Run_Time_Counter,0,8)OTU(Port_Data.Port_Read.[Port])OTL(Local_Control.6);
   55: NOP();
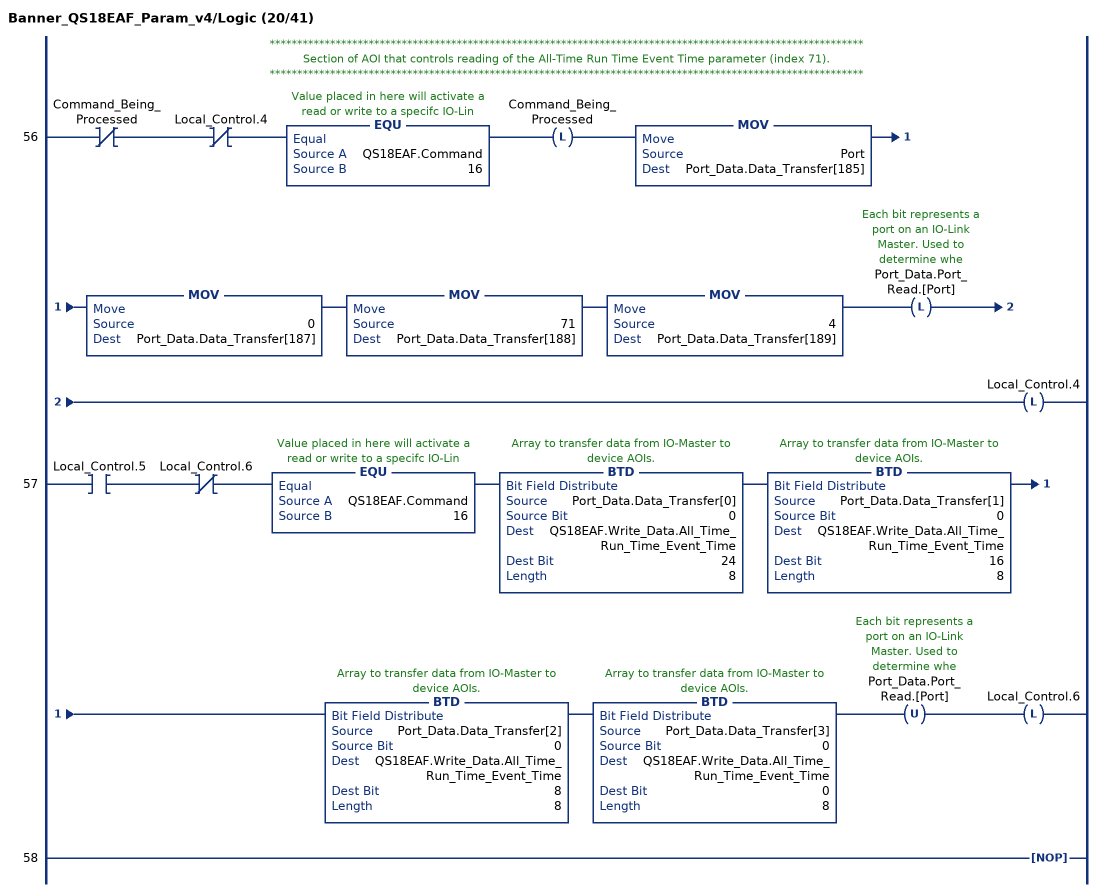
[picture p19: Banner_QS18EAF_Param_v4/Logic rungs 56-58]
   // ************************************************************************************************************
   // Section of AOI that controls reading of the All-Time Run Time Event Time parameter (index 71).
   // ************************************************************************************************************
   56: XIO(Command_Being_Processed)XIO(Local_Control.4)EQU(QS18EAF.Command,16)OTL(Command_Being_Processed)MOV(Port,Port_Data.Data_Transfer[185])MOV(0,Port_Data.Data_Transfer[187])MOV(71,Port_Data.Data_Transfer[188])MOV(4,Port_Data.Data_Transfer[189])OTL(Port_Data.Port_Read.[Port])OTL(Local_Control.4);
   57: XIC(Local_Control.5)XIO(Local_Control.6)EQU(QS18EAF.Command,16)BTD(Port_Data.Data_Transfer[0],0,QS18EAF.Write_Data.All_Time_Run_Time_Event_Time,24,8)BTD(Port_Data.Data_Transfer[1],0,QS18EAF.Write_Data.All_Time_Run_Time_Event_Time,16,8)BTD(Port_Data.Data_Transfer[2],0,QS18EAF.Write_Data.All_Time_Run_Time_Event_Time,8,8)BTD(Port_Data.Data_Transfer[3],0,QS18EAF.Write_Data.All_Time_Run_Time_Event_Time,0,8)OTU(Port_Data.Port_Read.[Port])OTL(Local_Control.6);
   58: NOP();
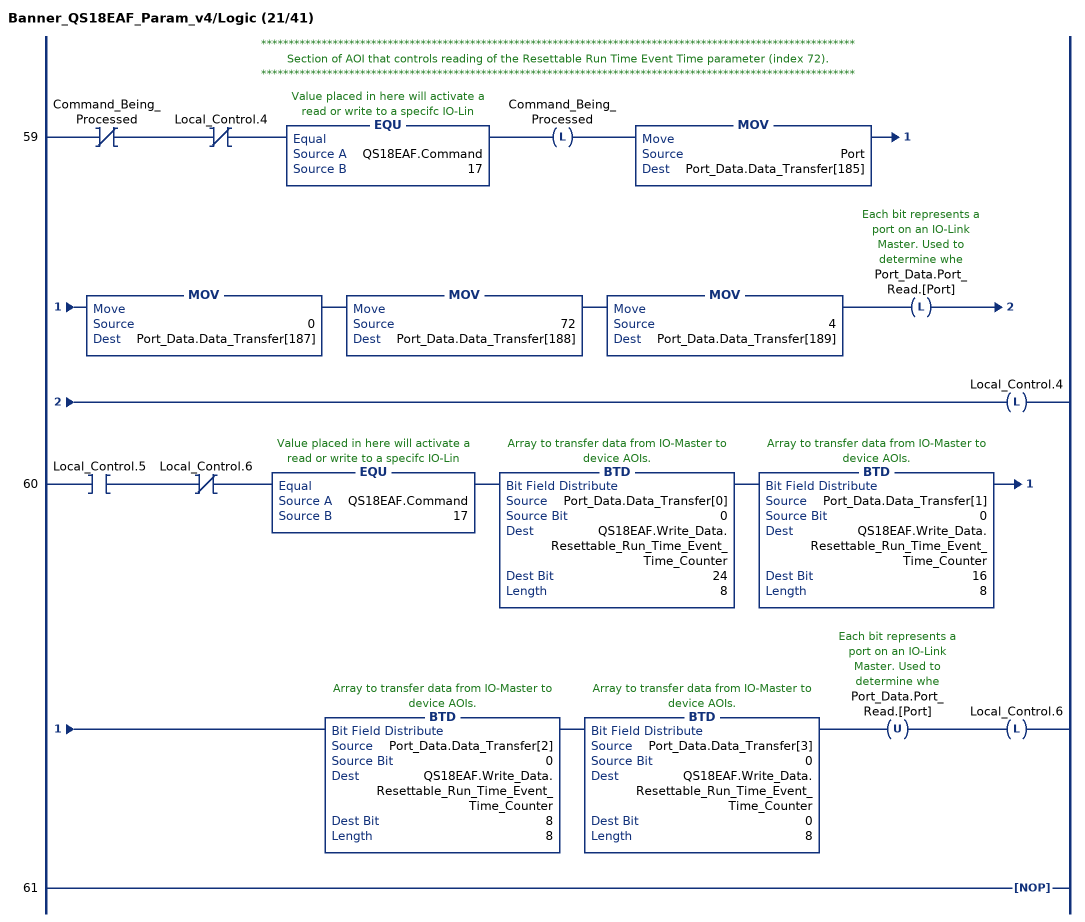
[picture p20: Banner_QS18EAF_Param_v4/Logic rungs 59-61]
   // ************************************************************************************************************
   // Section of AOI that controls reading of the Resettable Run Time Event Time parameter (index 72).
   // ************************************************************************************************************
   59: XIO(Command_Being_Processed)XIO(Local_Control.4)EQU(QS18EAF.Command,17)OTL(Command_Being_Processed)MOV(Port,Port_Data.Data_Transfer[185])MOV(0,Port_Data.Data_Transfer[187])MOV(72,Port_Data.Data_Transfer[188])MOV(4,Port_Data.Data_Transfer[189])OTL(Port_Data.Port_Read.[Port])OTL(Local_Control.4);
   60: XIC(Local_Control.5)XIO(Local_Control.6)EQU(QS18EAF.Command,17)BTD(Port_Data.Data_Transfer[0],0,QS18EAF.Write_Data.Resettable_Run_Time_Event_Time_Counter,24,8)BTD(Port_Data.Data_Transfer[1],0,QS18EAF.Write_Data.Resettable_Run_Time_Event_Time_Counter,16,8)BTD(Port_Data.Data_Transfer[2],0,QS18EAF.Write_Data.Resettable_Run_Time_Event_Time_Counter,8,8)BTD(Port_Data.Data_Transfer[3],0,QS18EAF.Write_Data.Resettable_Run_Time_Event_Time_Counter,0,8)OTU(Port_Data.Port_Read.[Port])OTL(Local_Control.6);
   61: NOP();
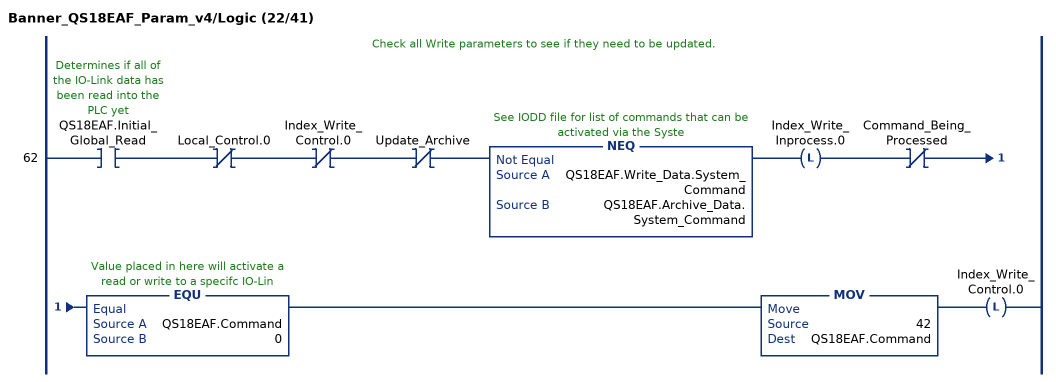
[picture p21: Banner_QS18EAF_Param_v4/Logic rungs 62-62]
   // Check all Write parameters to see if they need to be updated.
   62: XIC(QS18EAF.Initial_Global_Read)XIO(Local_Control.0)XIO(Index_Write_Control.0)XIO(Update_Archive)NEQ(QS18EAF.Write_Data.System_Command,QS18EAF.Archive_Data.System_Command)OTL(Index_Write_Inprocess.0)XIO(Command_Being_Processed)EQU(QS18EAF.Command,0)MOV(42,QS18EAF.Command)OTL(Index_Write_Control.0);
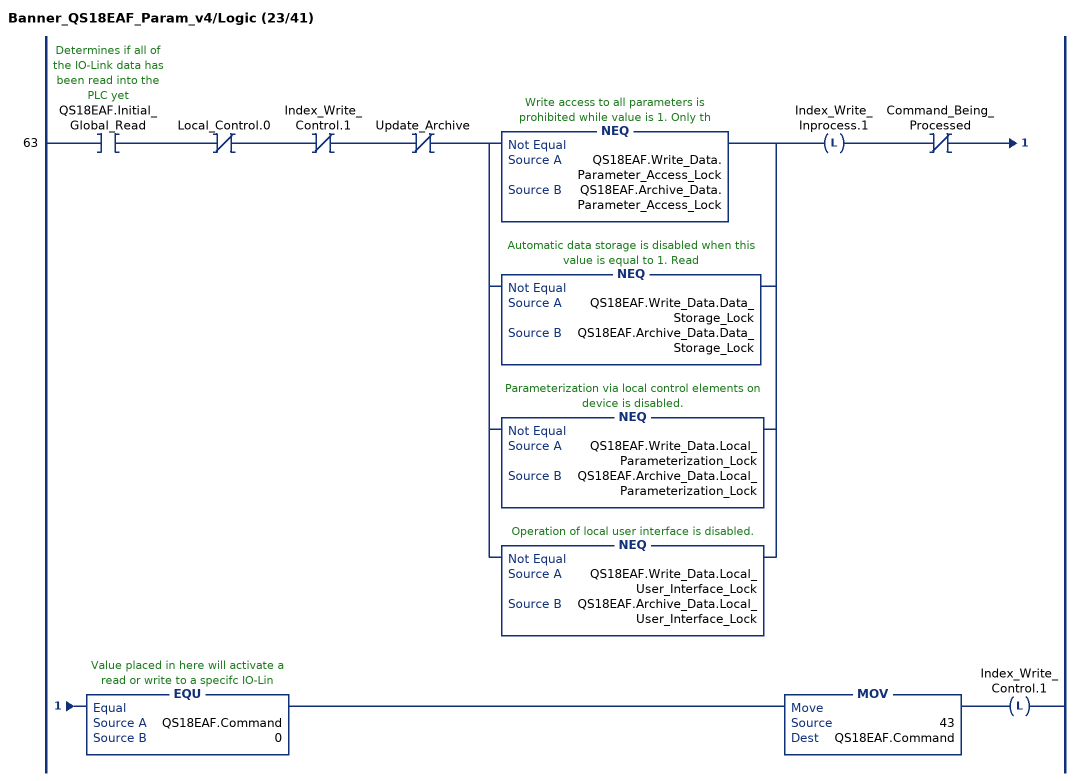
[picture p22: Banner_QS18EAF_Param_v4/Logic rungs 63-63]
   63: XIC(QS18EAF.Initial_Global_Read)XIO(Local_Control.0)XIO(Index_Write_Control.1)XIO(Update_Archive)[NEQ(QS18EAF.Write_Data.Parameter_Access_Lock,QS18EAF.Archive_Data.Parameter_Access_Lock) ,NEQ(QS18EAF.Write_Data.Data_Storage_Lock,QS18EAF.Archive_Data.Data_Storage_Lock) ,NEQ(QS18EAF.Write_Data.Local_Parameterization_Lock,QS18EAF.Archive_Data.Local_Parameterization_Lock) ,NEQ(QS18EAF.Write_Data.Local_User_Interface_Lock,QS18EAF.Archive_Data.Local_User_Interface_Lock) ]OTL(Index_Write_Inprocess.1)XIO(Command_Being_Processed)EQU(QS18EAF.Command,0)MOV(43,QS18EAF.Command)OTL(Index_Write_Control.1);
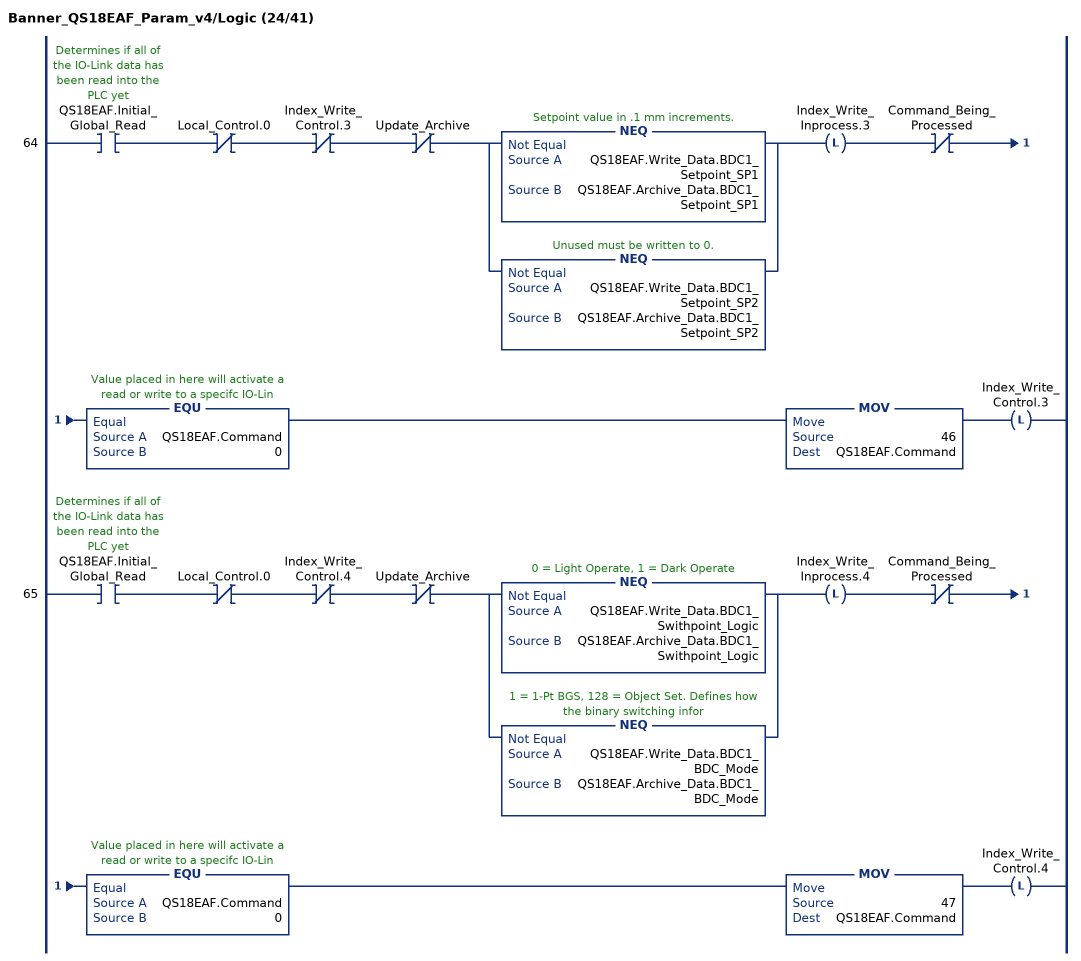
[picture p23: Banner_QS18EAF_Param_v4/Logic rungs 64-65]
   64: XIC(QS18EAF.Initial_Global_Read)XIO(Local_Control.0)XIO(Index_Write_Control.3)XIO(Update_Archive)[NEQ(QS18EAF.Write_Data.BDC1_Setpoint_SP1,QS18EAF.Archive_Data.BDC1_Setpoint_SP1) ,NEQ(QS18EAF.Write_Data.BDC1_Setpoint_SP2,QS18EAF.Archive_Data.BDC1_Setpoint_SP2) ]OTL(Index_Write_Inprocess.3)XIO(Command_Being_Processed)EQU(QS18EAF.Command,0)MOV(46,QS18EAF.Command)OTL(Index_Write_Control.3);
   65: XIC(QS18EAF.Initial_Global_Read)XIO(Local_Control.0)XIO(Index_Write_Control.4)XIO(Update_Archive)[NEQ(QS18EAF.Write_Data.BDC1_Swithpoint_Logic,QS18EAF.Archive_Data.BDC1_Swithpoint_Logic) ,NEQ(QS18EAF.Write_Data.BDC1_BDC_Mode,QS18EAF.Archive_Data.BDC1_BDC_Mode) ]OTL(Index_Write_Inprocess.4)XIO(Command_Being_Processed)EQU(QS18EAF.Command,0)MOV(47,QS18EAF.Command)OTL(Index_Write_Control.4);
